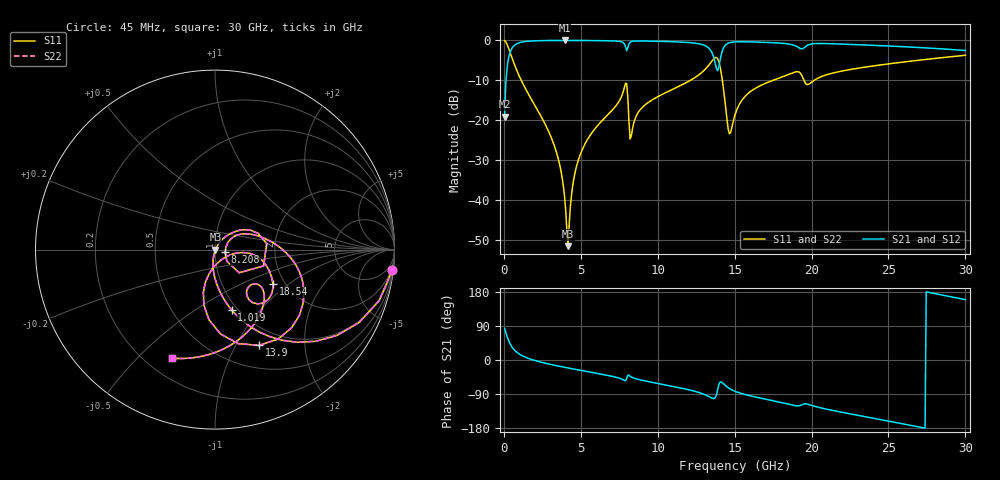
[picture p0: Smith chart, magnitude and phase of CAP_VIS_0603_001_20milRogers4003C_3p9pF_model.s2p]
! S-parameter model data by Modelithics Inc.  support@modelithics.com  813-866-6335  Tampa FL USA
! S-Parameter data specifications:
! Substrate: 20-mil Rogers 4003C, substrate thickness, H=0.508mm, Dielectric constant, Er=3.75
! PCB Mounting Pad Footprint: Pad width, PadW=0.90mm , Pad length, PadL=1.00mm , Pad gap, PadG (edge-to-edge)=1.00mm , Reference planes=3.0mm apart
! Created Wed Nov 18 13:22:21 2015
# hz S ma R 50
! 2 Port Network Data from SP1.SP block
! freq  magS11  angS11  magS21  angS21  magS12  angS12  magS22  angS22
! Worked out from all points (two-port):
!   401 points, 45 MHz to 30 GHz, reference 50 ohm
!   highest |S21| = -0.03 dB at 3.939 GHz (marker M1); lowest = -19.1 dB at 45 MHz (marker M2)
!   |S21| within 3 dB of the highest: 401.9 MHz to 13.52 GHz (13.12 GHz wide, 188 % of centre); 14.17 GHz to end of sweep
!   lowest |S11| = -51.6 dB at 4.164 GHz (marker M3), VSWR 1.01, Z = 50.3 - j0.066 ohm
!   |S11| at or under -10 dB: 1.125 GHz to 12.13 GHz (11 GHz wide, 166 % of centre); 14.2 GHz to 17.5 GHz (3.304 GHz wide, 20.8 % of centre); 19.5 GHz to 20.17 GHz (674.2 MHz wide, 3.4 % of centre)
!   |S22| runs from -51.6 to -0.1 dB; largest |S21 - S12| = 0
!   S11 on the Smith chart (normalised r, x): 45 MHz: 1, -17; 1.019 GHz: 0.94, -0.72; 8.208 GHz: 1.12, -0.03; 13.9 GHz: 0.77, -1.25; 18.54 GHz: 1.73, -0.78; 30 GHz: 0.30, -0.64
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4.5e7  0.9938 -6.6  0.1108 83.4  0.1108 83.4  0.9938 -6.6
3.4455e8  0.7584 -42.4  0.6513 47.6  0.6513 47.6  0.7584 -42.4
1.018538e9  0.3497 -74.5  0.9356 15.3  0.9356 15.3  0.3497 -74.5
3.190275e9  0.05332 -100.6  0.996 -13.0  0.996 -13.0  0.05332 -100.6
3.93915e9  0.0112 -96.1  0.9971 -19.2  0.9971 -19.2  0.0112 -96.1
4.163812e9  0.002644 -14.4  0.997 -21.0  0.997 -21.0  0.002644 -14.4
4.613138e9  0.0216 58.1  0.9966 -24.5  0.9966 -24.5  0.0216 58.1
5.062462e9  0.04145 58.0  0.9957 -27.9  0.9957 -27.9  0.04145 58.0
7.8333e9  0.2568 20.6  0.8991 -53.8  0.8991 -53.8  0.2568 20.6
8.207738e9  0.0583 -14.4  0.9477 -43.0  0.9477 -43.0  0.0583 -14.4
1.007992e10  0.2007 25.9  0.9728 -62.4  0.9728 -62.4  0.2007 25.9
1.285076e10  0.3944 -2.3  0.8898 -88.1  0.8898 -88.1  0.3944 -2.3
1.359964e10  0.5743 -31.1  0.6475 -101.6  0.6475 -101.6  0.5743 -31.1
1.389919e10  0.5874 -65.3  0.4169 -77.5  0.4169 -77.5  0.5874 -65.3
1.419874e10  0.316 -101.3  0.7398 -59.8  0.7398 -59.8  0.316 -101.3
1.464806e10  0.0678 -62.5  0.9324 -75.1  0.9324 -75.1  0.0678 -62.5
1.50225e10  0.1163 -10.2  0.9571 -82.5  0.9571 -82.5  0.1163 -10.2
1.599604e10  0.2259 -8.3  0.9568 -94.3  0.9568 -94.3  0.2259 -8.3
1.854221e10  0.3758 -31.0  0.8978 -116.8  0.8978 -116.8  0.3758 -31.0
2.003996e10  0.3031 -39.4  0.9043 -120.3  0.9043 -120.3  0.3031 -39.4
2.505742e10  0.509 -72.6  0.8491 -161.7  0.8491 -161.7  0.509 -72.6
3e10  0.6507 -111.5  0.746 159.3  0.746 159.3  0.6507 -111.5
